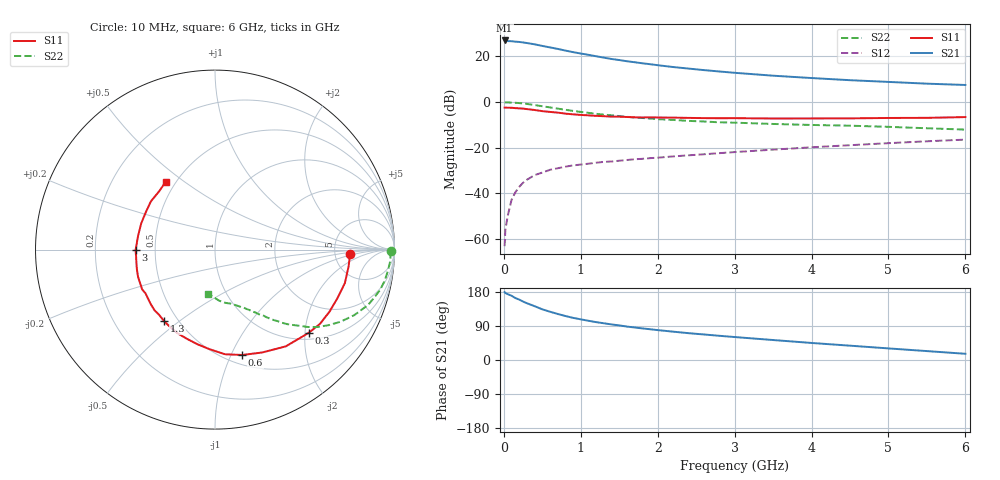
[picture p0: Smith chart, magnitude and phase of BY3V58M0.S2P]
! SIEMENS Small Signal Semiconductors
! BFY420
! Si NPN RF SIEGET Grounded Emitter Transistor in MICRO-X
! VCE = 3.5 V  IC = 8 mA
! Common Emitter S-Parameters:  October  1996
# GHz  S  MA  R  50
!  f  S11  S21  S12  S22
! GHz  MAG  ANG  MAG  ANG  MAG  ANG  MAG  ANG
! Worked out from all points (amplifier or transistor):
!   36 points, 10 MHz to 6 GHz, reference 50 ohm
!   highest |S21| = 26.9 dB at 10 MHz (marker M1)
!   |S21| within 3 dB of that: start of sweep to 594.3 MHz
!   unconditionally stable (mu >= 1): start of sweep to 10.55 MHz; 2.708 GHz to end of sweep
!   at 250 MHz: K = 0.19, MSG = 30.7 dB, |S12| = -35.3 dB
!   at 1.4 GHz: K = 0.68, MSG = 22.4 dB, |S12| = -26.0 dB
!   at 6 GHz: K = 1.10, MAG = 10.0 dB, |S12| = -16.5 dB
!   S11 on the Smith chart (normalised r, x): 10 MHz: 6.97, -0.76; 300 MHz: 1.16, -2.10; 600 MHz: 0.59, -1.10; 1.3 GHz: 0.42, -0.44; 3 GHz: 0.39, -0.00; 6 GHz: 0.44, +0.43
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0.01  0.7518 -1.8  22.21 179.2  0.0007 51.2  0.9783 -0.6
0.02  0.7519 -3.3  22 176.8  0.0016 64.6  0.9769 -1.3
0.05  0.7502 -7.1  21.54 173.8  0.0032 79.4  0.9794 -3.4
0.1  0.7473 -14.4  21.36 169.6  0.0072 78.8  0.9707 -7.0
0.15  0.7341 -21.6  20.92 163.5  0.0106 76.7  0.9607 -10.5
0.2  0.7256 -28.5  20.61 159.4  0.0139 74.9  0.9472 -13.7
0.25  0.7164 -35.3  20.1 154.2  0.0171 70.8  0.9255 -16.9
0.3  0.6987 -41.5  19.5 149.8  0.0199 69.8  0.9068 -19.9
0.4  0.668 -53.8  18.29 142.0  0.0251 64.8  0.8576 -25.2
0.5  0.6305 -65.4  16.86 133.7  0.0286 60.7  0.8077 -29.8
0.6  0.6064 -75.5  15.66 127.4  0.0328 57.6  0.7608 -33.6
0.8  0.5561 -93.0  13.34 116.1  0.0384 52.1  0.6754 -39.7
0.9  0.5368 -100.3  12.33 111.2  0.041 50.7  0.6382 -41.8
1.1  0.5101 -114.6  10.76 103.5  0.0447 49.5  0.5784 -45.9
1.3  0.4891 -125.4  9.35 96.9  0.0489 47.6  0.5295 -48.8
1.7  0.4622 -143.8  7.417 85.8  0.0558 46.6  0.4577 -53.6
2.2  0.4548 -160.5  5.823 74.8  0.0644 45.7  0.4051 -58.6
3  0.4427 -179.6  4.354 60.6  0.0801 44.0  0.353 -65.3
3.5  0.4353 169.7  3.763 52.7  0.0907 42.4  0.3306 -69.5
4.5  0.4382 151.7  3 37.8  0.1135 37.4  0.3031 -78.6
5.5  0.45 133.6  2.518 23.5  0.1381 30.7  0.2663 -91.2
6  0.4674 125.9  2.357 16.4  0.1504 26.6  0.2487 -99.2
